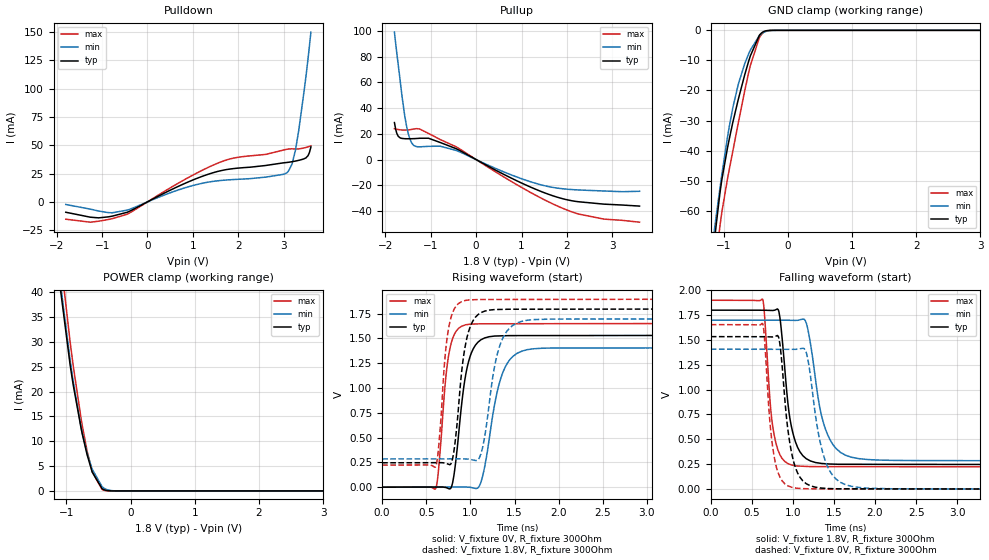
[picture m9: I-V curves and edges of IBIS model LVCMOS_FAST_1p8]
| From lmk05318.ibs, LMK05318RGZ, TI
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|   LVCMOS_FAST_1p8V Model
[Model]   LVCMOS_FAST_1p8
Model_type   3-state
Polarity   Non-Inverting
Vmeas = 0.9
Vref = 0
Cref = 2pF
Rref = 100000
|   typ   min   max
C_comp   1.5263E-12   1.43105E-12   1.63546E-12
| Where nom  PVT is Nominal Process, 1.8V, 27C
|   Fast PVT is Strong Process,  1.9V, -40C
|   Slow PVT is Weak Process,   1.7V, 125C
[Voltage Range]   1.8   1.7   1.9
|Junction Temperature
[Temperature Range]   27   125   -40
[Pullup Reference]   1.8   1.7   1.9
[Pulldown Reference]   0   0   -0
[Power Clamp Reference]   1.8   1.7   1.9
[GND Clamp Reference]   0   0   0
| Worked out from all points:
|   slope of the pulldown table from 0 to 0.27 V, typ, clamps not added: 47.6 ohm
|   slope of the pullup table from 0 to 0.27 V, typ, clamps not added: 52 ohm
|   GND clamp passes 1 mA (typ) near -0.42 V on its own axis
|   POWER clamp passes 1 mA (typ) near -0.47 V on its own axis
|   falling waveform, V_fixture 1.8V, R_fixture 300Ohm: 20-80 % time 130ps typ, 190ps min, 99.8ps max; typ from 1.8 V to 0.247 V
|   rising waveform, V_fixture 0V, R_fixture 300Ohm: 20-80 % time 128ps typ, 177ps min, 98.4ps max; typ from 0 V to 1.53 V
|   rising waveform, V_fixture 1.8V, R_fixture 300Ohm: 20-80 % time 116ps typ, 156ps min, 91ps max; typ from 0.246 V to 1.8 V
|   falling waveform, V_fixture 0V, R_fixture 300Ohm: 20-80 % time 130ps typ, 180ps min, 102ps max; typ from 1.53 V to 0.001 V
[Pulldown]
|   Voltage   I(typ)   I(min)   I(max)
-1.8V     -9.189mA   -2.317mA   -15.34mA
-1.26V    -13.55mA   -6.429mA   -17.98mA
-779.4mV  -12.68mA   -9.656mA   -14.92mA
-444.6mV  -9.188mA   -7.294mA   -10.91mA
765mV     15.27mA    11.65mA    18.48mA
1.58V     27.23mA    18.77mA    34.74mA
3.071V    34.82mA    25.76mA    46.52mA
3.179V    35.46mA    32.99mA    46.89mA
3.26V     36.08mA    45.72mA    46.75mA
3.438V    37.89mA    94.45mA    47.56mA
3.535V    40.78mA    126mA      48.62mA
3.6V      48.48mA    150.1mA    49.52mA
[GND Clamp]
|   Voltage   I(typ)   I(min)   I(max)
-1.8V     -222mA     -232.5mA   -284.8mA
-1.13V    -67.53mA   -64.1mA    -78.56mA
-1.12V    -65.36mA   -62.34mA   -76.36mA
-1.055V   -53.69mA   -52.05mA   -64.62mA
-909mV    -35.8mA    -31.61mA   -45.9mA
-768.6mV  -22.68mA   -17.68mA   -30.43mA
-671.4mV  -14.76mA   -11.07mA   -20.07mA
-585mV    -8.557mA   -6.603mA   -11.77mA
-444.6mV  -1.689mA   -1.773mA   -2.479mA
-385.2mV  -510.1uA   -771.6uA   -829.2uA
-217.8mV  -3.668uA   -26.55uA   -3.586uA
3.6V      0A         0A         0A
[Pullup]
|   Voltage   I(typ)   I(min)   I(max)
-1.8V     28.83mA    99.08mA    24.02mA
-1.751V   20.89mA    83.98mA    23.62mA
-1.714V   18.08mA    73.01mA    23.38mA
-1.568V   16.3mA     32.99mA    22.97mA
-1.465V   16.26mA    16.65mA    23.22mA
-1.373V   16.34mA    11.04mA    23.83mA
-1.049V   16.66mA    10.35mA    20.4mA
-444.6mV  8.615mA    7.24mA     10.08mA
991.8mV   -17.98mA   -14.67mA   -21.36mA
1.937V    -30.58mA   -22.69mA   -38.19mA
2.817V    -34.52mA   -24.32mA   -46.15mA
3.6V      -36.04mA   -24.53mA   -48.54mA
[POWER Clamp]
|   Voltage   I(typ)   I(min)   I(max)
-1.8V     160.9mA    273.9mA    172.1mA
-1.098V   41.18mA    42.33mA    47.69mA
-941.4mV  25.34mA    26.35mA    29.98mA
-892.8mV  21.3mA     22.01mA    25.16mA
-768.6mV  12.47mA    12.68mA    14.38mA
-752.4mV  11.47mA    11.67mA    13.15mA
-676.8mV  7.278mA    7.609mA    8.016mA
-595.8mV  3.769mA    4.329mA    3.814mA
-444.6mV  458.7uA    874.5uA    303.3uA
-352.8mV  57.31uA    198.4uA    23.38uA
-217.8mV  990.9nA    11.87uA    113.1nA
3.6V      0A         0A         0A
[Ramp]
R_load = 300
|   typ   min   max
dV/dt_r   0.918258/1.27829e-10   0.842774/1.77161e-10   0.99065/9.83516e-11
dV/dt_f   0.930078/1.30292e-10   0.846501/1.89839e-10   1.00374/9.97727e-11
[Falling Waveform]
V_fixture = 1.8V
V_fixture_min = 1.7V
V_fixture_max = 1.9V
R_fixture = 300Ohm
C_fixture = 0F
|   Time   V(typ)   V(min)   V(max)
0s        1.797V     1.697V     1.896V
633.3ps   1.796V     1.696V     1.901V
759.4ps   1.794V     1.696V     602.9mV
840.9ps   1.728V     1.696V     346.8mV
942.5ps   839.5mV    1.695V     255.7mV
1.032ns   473.3mV    1.694V     235.7mV
1.152ns   313.9mV    1.69V      229.3mV
1.366ns   257.4mV    681.3mV    227mV
1.642ns   250.2mV    340.7mV    226.7mV
5ns       246.5mV    285.7mV    223.2mV
[Rising Waveform]
V_fixture = 0V
V_fixture_min = 0V
V_fixture_max = 0V
R_fixture = 300Ohm
C_fixture = 0F
|   Time   V(typ)   V(min)   V(max)
0s        255.4uV    550.4uV    90.53uV
609.1ps   1.471mV    1.278mV    -8.102mV
748.3ps   -12.73mV   1.444mV    1.302V
811.8ps   111.1mV    1.52mV     1.527V
901.5ps   842.7mV    1.627mV    1.623V
978.4ps   1.264V     44.41uV    1.641V
1.085ns   1.462V     -6.083mV   1.646V
1.344ns   1.525V     1.099V     1.647V
1.582ns   1.528V     1.371V     1.647V
5ns       1.531V     1.405V     1.651V
[Rising Waveform]
V_fixture = 1.8V
V_fixture_min = 1.7V
V_fixture_max = 1.9V
R_fixture = 300Ohm
C_fixture = 0F
|   Time   V(typ)   V(min)   V(max)
0s        246mV      285.1mV    222.7mV
609.1ps   247mV      285.5mV    212.6mV
748.3ps   232.4mV    285.6mV    1.579V
811.8ps   355.7mV    285.6mV    1.786V
901.5ps   1.169V     285.7mV    1.871V
978.4ps   1.566V     282.9mV    1.886V
1.118ns   1.758V     332.2mV    1.891V
1.307ns   1.791V     1.349V     1.892V
1.528ns   1.793V     1.654V     1.892V
5ns       1.796V     1.696V     1.896V
[Falling Waveform]
|Gnd
V_fixture = 0V
V_fixture_min = 0V
V_fixture_max = 0V
R_fixture = 300Ohm
C_fixture = 0F
|   Time   V(typ)   V(min)   V(max)
0s        1.531V     1.405V     1.651V
633.3ps   1.53V      1.404V     1.658V
759.4ps   1.529V     1.404V     388.8mV
840.9ps   1.461V     1.404V     122.9mV
942.5ps   575.5mV    1.404V     32.1mV
1.032ns   214.5mV    1.404V     12.34mV
1.152ns   62.5mV     1.395V     5.281mV
1.366ns   10.36mV    358mV      3.436mV
1.642ns   3.925mV    44.98mV    2.991mV
5ns       679.9uV    1.04mV     531.2uV
